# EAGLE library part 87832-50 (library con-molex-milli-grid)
HEADER
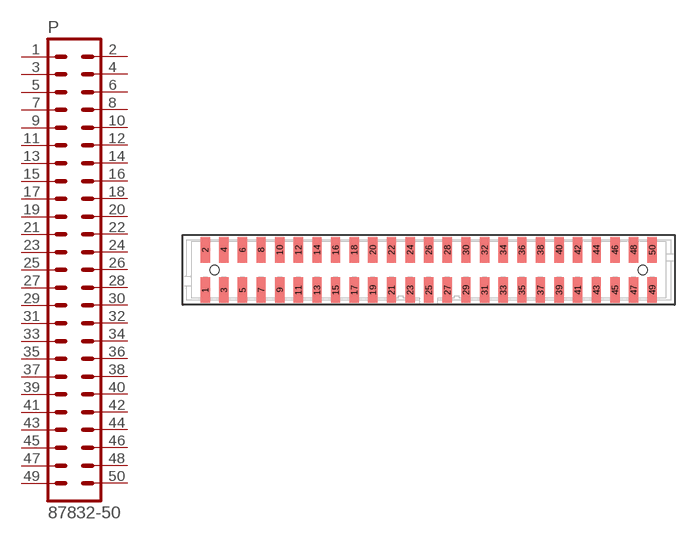
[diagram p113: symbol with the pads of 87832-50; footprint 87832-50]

Designator prefix P

## 87832-50  [87832-50]
1  1  pas
2  2  pas
3  3  pas
4  4  pas
5  5  pas
6  6  pas
7  7  pas
8  8  pas
9  9  pas
10  10  pas
11  11  pas
12  12  pas
13  13  pas
14  14  pas
15  15  pas
16  16  pas
17  17  pas
18  18  pas
19  19  pas
20  20  pas
21  21  pas
22  22  pas
23  23  pas
24  24  pas
25  25  pas
26  26  pas
27  27  pas
28  28  pas
29  29  pas
30  30  pas
31  31  pas
32  32  pas
33  33  pas
34  34  pas
35  35  pas
36  36  pas
37  37  pas
38  38  pas
39  39  pas
40  40  pas
41  41  pas
42  42  pas
43  43  pas
44  44  pas
45  45  pas
46  46  pas
47  47  pas
48  48  pas
49  49  pas
50  50  pas

## Footprint 87832-50 (pad centres in mm)
HEADER SMD Dual Row, Shrouded, Vertical
smd 1 x 2.75: 1 -24,-2.15; 2 -24,2.15; 3 -22,-2.15; 4 -22,2.15; 5 -20,-2.15; 6 -20,2.15; 7 -18,-2.15; 8 -18,2.15; 9 -16,-2.15; 10 -16,2.15; 11 -14,-2.15; 12 -14,2.15; 13 -12,-2.15; 14 -12,2.15; 15 -10,-2.15; 16 -10,2.15; 17 -8,-2.15; 18 -8,2.15; 19 -6,-2.15; 20 -6,2.15; 21 -4,-2.15; 22 -4,2.15; 23 -2,-2.15; 24 -2,2.15; 25 0,-2.15; 26 0,2.15; 27 2,-2.15; 28 2,2.15; 29 4,-2.15; 30 4,2.15; 31 6,-2.15; 32 6,2.15; 33 8,-2.15; 34 8,2.15; 35 10,-2.15; 36 10,2.15; 37 12,-2.15; 38 12,2.15; 39 14,-2.15; 40 14,2.15; 41 16,-2.15; 42 16,2.15; 43 18,-2.15; 44 18,2.15; 45 20,-2.15; 46 20,2.15; 47 22,-2.15; 48 22,2.15; 49 24,-2.15; 50 24,2.15
hole 1 at -23,0
hole 1 at 23,0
